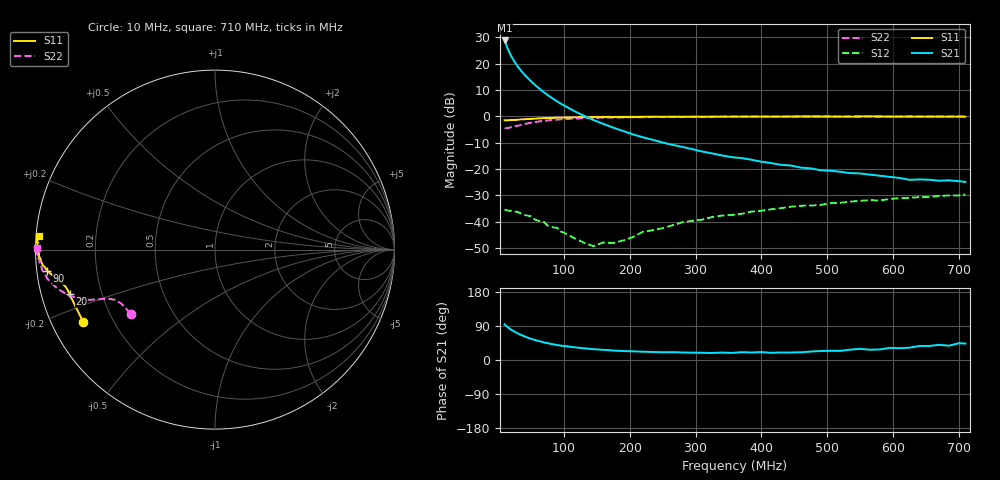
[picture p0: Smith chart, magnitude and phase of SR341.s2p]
!  POLYFET RF DEVICES
!  SR341  (Each side)
!  S PARAMETERS
!  VDS=50V, IDQ=400mA
# MHZ S MA R 50
! Freq=Mhz Mag[s11] Ang[s11] Mag[s21] Ang[s21] Mag[s12] Ang[s12] Mag[s22] Ang[s22]
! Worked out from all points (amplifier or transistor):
!   60 points, 10 MHz to 710 MHz, reference 50 ohm
!   highest |S21| = 28.8 dB at 10 MHz (marker M1)
!   |S21| within 3 dB of that: start of sweep to 14.54 MHz
!   unconditionally stable (mu >= 1): nowhere
!   at 60 MHz: K = 0.16, MSG = 25.3 dB, |S12| = -39.5 dB
!   at 280 MHz: K = 0.51, MSG = 14.3 dB, |S12| = -40.2 dB
!   at 710 MHz: K = 0.96, MSG = 2.4 dB, |S12| = -29.7 dB
!   S11 on the Smith chart (normalised r, x): 10 MHz: 0.09, -0.26; 20 MHz: 0.08, -0.15; 90 MHz: 0.03, -0.06; 710 MHz: 0.01, +0.04
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10  0.8375 -151.1  27.4 94.2  0.01705 8.7  0.5899 -142.8
15  0.8403 -158.6  18.73 85.9  0.01628 -1.0  0.6025 -150.0
20  0.8472 -162.9  13.81 79.8  0.01616 -5.9  0.6206 -153.2
25  0.8529 -165.2  10.86 74.8  0.01559 -12.6  0.6421 -154.6
30  0.8626 -166.7  8.804 70.2  0.01546 -14.1  0.6632 -155.6
35  0.873 -167.7  7.319 66.3  0.01422 -15.2  0.6866 -156.5
40  0.8789 -168.3  6.202 62.5  0.01355 -21.8  0.7113 -156.9
45  0.8878 -168.9  5.331 59.1  0.0131 -22.1  0.7343 -157.7
50  0.8945 -169.6  4.627 56.0  0.01266 -23.4  0.7538 -158.2
55  0.903 -170.1  4.043 53.4  0.0112 -24.5  0.7723 -159.0
65  0.9154 -170.9  3.175 48.6  0.01003 -27.7  0.8077 -160.4
75  0.9264 -171.8  2.549 44.4  0.0085 -28.1  0.8326 -161.6
90  0.9421 -172.7  1.907 39.5  0.0077 -29.2  0.8674 -163.7
115  0.9543 -174.2  1.271 33.7  0.00494 -22.0  0.9044 -166.1
130  0.9637 -174.8  1.031 31.0  0.00405 -8.6  0.919 -167.4
145  0.9658 -175.4  0.8505 28.5  0.00345 15.3  0.9306 -168.6
175  0.9723 -176.7  0.609 24.9  0.00396 34.7  0.9492 -170.4
250  0.9802 -178.4  0.3186 20.5  0.00758 81.4  0.9706 -173.6
370  0.9856 179.8  0.1614 20.5  0.01418 91.9  0.9804 -176.2
490  0.9909 178.3  0.09499 23.6  0.02087 95.4  0.9873 -178.2
595  0.9871 176.7  0.07101 32.0  0.02706 96.9  0.988 -179.6
710  0.9853 175.6  0.05697 43.3  0.03291 100.1  0.9916 179.4
